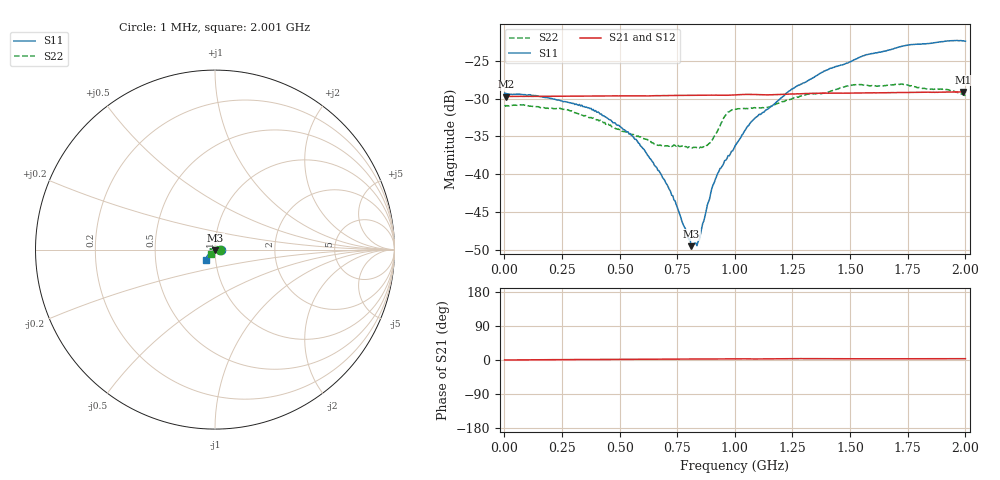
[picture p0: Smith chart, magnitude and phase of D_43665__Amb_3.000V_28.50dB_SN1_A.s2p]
! device id: 43665_
! dir: \\malibu\benchdata\1_engineers\tn_data\43665_75ohm\new\sparar\43665_\amb\3p000v\28p50db
! Serial: 1
! Insertion: A
! Temp: Amb
! VDD: 3.000V
! Attenuation Step: 28.50dB
! IDD: 1.452462e+00mA
! FILE NAME
! DATE 03-27-2009 08:40:23
! CORRECTED  DATA
#  Hz  S  RI  R  75
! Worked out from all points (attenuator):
!   401 points, 1 MHz to 2.001 GHz, reference 75 ohm
!   highest |S21| = -29.11 dB at 1.991 GHz (marker M1); lowest = -29.7 dB at 6 MHz (marker M2)
!   lowest |S11| = -49.5 dB at 811 MHz (marker M3), VSWR 1.01, Z = 75.3 - j0.427 ohm
!   |S11| at or under -10 dB: start of sweep to end of sweep
!   |S22| runs from -36.5 to -28.1 dB; largest |S21 - S12| = 0.00026
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1000000  0.0344 -0.000316  0.0329 0.000132  0.0327 0.000192  0.0287 -0.000221
6000000  0.0342 -0.00048  0.0326 7.79e-05  0.0328 -8.79e-05  0.0281 0.000171
2.41e8  0.0307 0.00197  0.0328 0.000548  0.0328 0.000575  0.0248 0.0116
3.36e8  0.0286 0.00215  0.0329 0.000714  0.0328 0.000758  0.0196 0.0149
4.06e8  0.0256 0.00295  0.0329 0.00089  0.0329 0.000944  0.0159 0.0164
5.46e8  0.0184 0.00177  0.033 0.00108  0.033 0.00111  0.0073 0.0171
6.71e8  0.0106 2.38e-05  0.0331 0.00141  0.0331 0.00143  -0.000958 0.0155
7.41e8  0.0065 -0.00145  0.0332 0.00141  0.0332 0.00153  -0.0051 0.0146
8.11e8  0.00177 -0.00283  0.0332 0.00148  0.0333 0.00157  -0.0103 0.0108
8.41e8  -9.88e-05 -0.0036  0.0333 0.00152  0.0333 0.0016  -0.0121 0.00896
8.81e8  -0.00354 -0.00516  0.0333 0.00149  0.0334 0.00163  -0.0144 0.00581
9.11e8  -0.00589 -0.00655  0.0333 0.00155  0.0333 0.00163  -0.0174 0.00362
9.61e8  -0.00911 -0.00841  0.0332 0.00168  0.0333 0.00182  -0.0245 0.00306
1.001e9  -0.0123 -0.00922  0.0334 0.00185  0.0334 0.00198  -0.0265 0.00429
1.096e9  -0.0199 -0.0135  0.0336 0.00163  0.0336 0.00173  -0.0275 -0.000188
1.241e9  -0.0294 -0.0205  0.0338 0.00211  0.0339 0.00224  -0.0301 -0.00851
1.336e9  -0.0345 -0.0259  0.0342 0.00208  0.0343 0.00222  -0.0316 -0.0132
1.521e9  -0.0439 -0.0369  0.0344 0.00193  0.0345 0.00205  -0.0324 -0.0219
1.671e9  -0.0483 -0.0456  0.0345 0.00195  0.0347 0.00209  -0.0297 -0.0248
1.916e9  -0.0508 -0.0564  0.0349 0.00207  0.035 0.00219  -0.0246 -0.0268
1.991e9  -0.0495 -0.0581  0.035 0.00211  0.0351 0.00212  -0.0214 -0.026
2.001e9  -0.0491 -0.0579  0.0349 0.0021  0.035 0.00213  -0.0211 -0.0255
